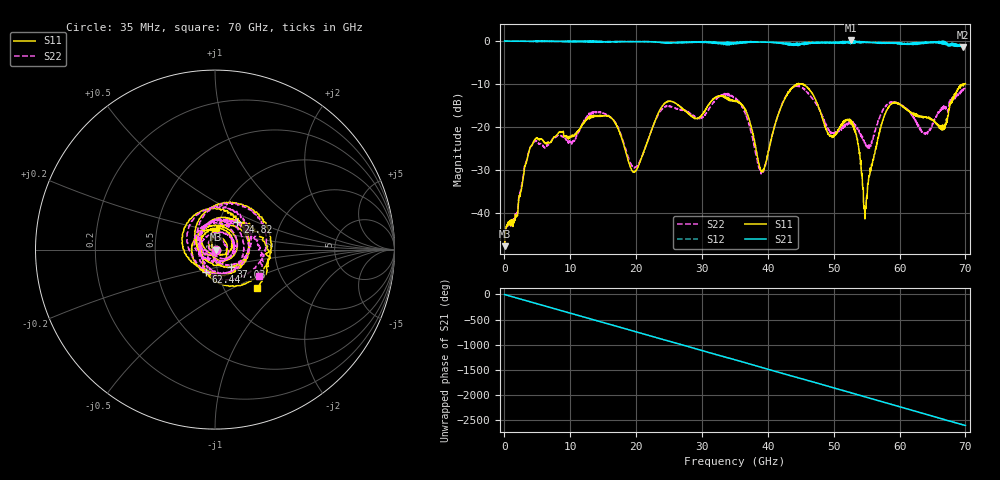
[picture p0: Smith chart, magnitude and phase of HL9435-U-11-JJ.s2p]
! 7/27/2020 10:51:02 AM
! H:\PRODUCTION_DATA\TEMP_S2P.S2P
! CHANNEL.1
! TR.MEASUREMENT
! CORRECTED.DATA
# GHZ S RI R 50.0
! FREQ.GHZ  S11RE  S11IM  S21RE  S21IM  S12RE  S12IM  S22RE  S22IM
!; PortSelection: Port_12
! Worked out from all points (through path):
!   2000 points, 35 MHz to 70 GHz, reference 50 ohm
!   highest |S21| = 0.08 dB at 52.64 GHz (marker M1); lowest = -1.4 dB at 69.61 GHz (marker M2)
!   group delay of S21, straight-line fit = 104 ps
!   lowest |S11| = -47.7 dB at 35 MHz (marker M3), VSWR 1.01, Z = 50.4 - j0.0276 ohm
!   |S11| at or under -10 dB: start of sweep to 44.48 GHz; 45.0632 GHz to 45.21641 GHz (153.2 MHz wide, 0.339 % of centre); 45.22 GHz to 69.89 GHz (24.66 GHz wide, 42.8 % of centre)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
!   |S22| runs from -47.6 to -10.3 dB; largest |S21 - S12| = 0.087
!   S11 on the Smith chart (normalised r, x): 35 MHz: 1.01, -0.00; 24.82 GHz: 1.21, +0.39; 37.03 GHz: 1.17, -0.23; 62.44 GHz: 0.88, -0.22; 70 GHz: 1.42, -0.68
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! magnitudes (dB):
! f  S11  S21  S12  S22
! 35 MHz  -47.7  0.0  0.0  -47.6
! 4.55 GHz  -23.1  -0.1  -0.1  -23.5
! 11.72 GHz  -19.7  -0.2  -0.1  -19.7
! 16.24 GHz  -17.9  -0.2  -0.2  -17.9
! 19.7 GHz  -30.5  -0.2  -0.2  -29.5
! 23.38 GHz  -16.8  -0.3  -0.3  -17.1
! 24.82 GHz  -14.0  -0.5  -0.5  -15.1
! 35.03 GHz  -13.9  -0.5  -0.5  -13.3
! 37.03 GHz  -17.7  -0.2  -0.3  -18.9
! 39.13 GHz  -30.5  -0.3  -0.3  -30.7
! 43.09 GHz  -12.0  -0.8  -0.9  -11.8
! 46.69 GHz  -12.0  -0.5  -0.4  -13.2
! 49.45 GHz  -22.1  -0.5  -0.4  -21.1
! 52.64 GHz  -18.9  0.1  -0.5  -19.3
! 53.66 GHz  -23.9  -0.2  -0.4  -20.6
! 54.77 GHz  -40.1  -0.4  -0.3  -23.6
! 58.34 GHz  -15.3  -0.6  -0.4  -14.5
! 62.44 GHz  -17.5  -0.8  -0.4  -18.8
! 64.08 GHz  -17.7  -0.3  -0.5  -21.5
! 66.75 GHz  -20.6  -0.4  -0.2  -15.7
! 69.61 GHz  -10.1  -1.4  -0.9  -11.6
! 70 GHz  -9.9  -1.1  -1.2  -10.9
